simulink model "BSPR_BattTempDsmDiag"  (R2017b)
settings: Solver=FixedStepDiscrete  StartTime=0.0  StopTime=10.0  FixedStep=1  RelTol=1e-3  EnableMultiTasking=on
libraries: simulink x112

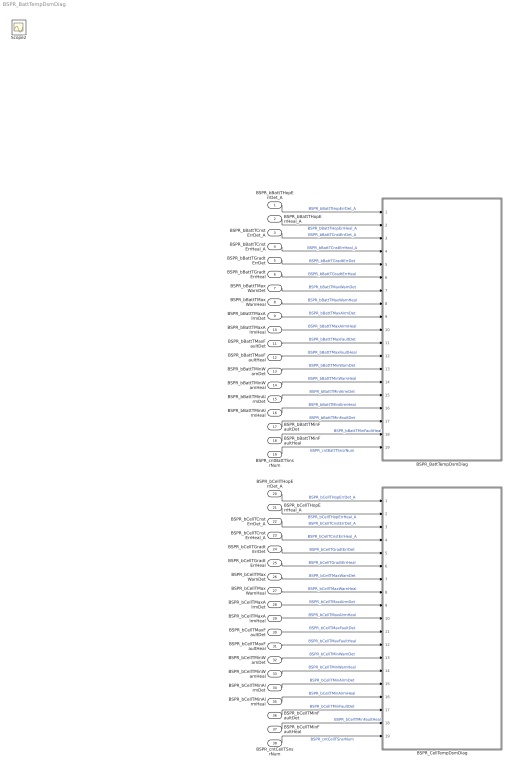
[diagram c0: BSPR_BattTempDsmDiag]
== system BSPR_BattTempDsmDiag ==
  BSPR_bBattTHopErrDet_A : Inport
  BSPR_bBattTHopErrHeal_A : Inport  Port=2
  BSPR_bBattTCnstErrDet_A : Inport  Port=3
  BSPR_bBattTCnstErrHeal_A : Inport  Port=4
  BSPR_bBattTGradtErrDet : Inport  Port=5  OutDataTypeStr=boolean
  BSPR_bBattTGradtErrHeal : Inport  Port=6  OutDataTypeStr=boolean
  BSPR_bBattTMaxWarnDet : Inport  Port=7
  BSPR_bBattTMaxWarnHeal : Inport  Port=8
  BSPR_bBattTMaxAlrmDet : Inport  Port=9
  BSPR_bBattTMaxAlrmHeal : Inport  Port=10
  BSPR_bBattTMaxFaultDet : Inport  Port=11
  BSPR_bBattTMaxFaultHeal : Inport  Port=12
  BSPR_bBattTMinWarnDet : Inport  Port=13
  BSPR_bBattTMinWarnHeal : Inport  Port=14
  BSPR_bBattTMinAlrmDet : Inport  Port=15
  BSPR_bBattTMinAlrmHeal : Inport  Port=16
  BSPR_bBattTMinFaultDet : Inport  Port=17
  BSPR_bBattTMinFaultHeal : Inport  Port=18
  BSPR_cntBattTSnsrNum : Inport  Port=19
  BSPR_bCellTHopErrDet_A : Inport  Port=20
  BSPR_bCellTHopErrHeal_A : Inport  Port=21
  BSPR_bCellTCnstErrDet_A : Inport  Port=22
  BSPR_bCellTCnstErrHeal_A : Inport  Port=23
  BSPR_bCellTGradtErrDet : Inport  Port=24  OutDataTypeStr=boolean
  BSPR_bCellTGradtErrHeal : Inport  Port=25  OutDataTypeStr=boolean
  BSPR_bCellTMaxWarnDet : Inport  Port=26
  BSPR_bCellTMaxWarnHeal : Inport  Port=27
  BSPR_bCellTMaxAlrmDet : Inport  Port=28
  BSPR_bCellTMaxAlrmHeal : Inport  Port=29
  BSPR_bCellTMaxFaultDet : Inport  Port=30
  BSPR_bCellTMaxFaultHeal : Inport  Port=31
  BSPR_bCellTMinWarnDet : Inport  Port=32
  BSPR_bCellTMinWarnHeal : Inport  Port=33
  BSPR_bCellTMinAlrmDet : Inport  Port=34
  BSPR_bCellTMinAlrmHeal : Inport  Port=35
  BSPR_bCellTMinFaultDet : Inport  Port=36
  BSPR_bCellTMinFaultHeal : Inport  Port=37
  BSPR_cntCellTSnsrNum : Inport  Port=38
  BSPR_BattTempDsmDiag : Subsystem
  BSPR_CellTempDsmDiag : Subsystem
  Scope2 : Scope
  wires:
  BSPR_bBattTMaxWarnDet/1 -> BSPR_BattTempDsmDiag/7(BSPR_bBattTMaxWarnDet)  "BSPR_bBattTMaxWarnDet"
  BSPR_bBattTMaxWarnHeal/1 -> BSPR_BattTempDsmDiag/8(BSPR_bBattTMaxWarnHeal)  "BSPR_bBattTMaxWarnHeal"
  BSPR_bBattTMaxAlrmDet/1 -> BSPR_BattTempDsmDiag/9(BSPR_bBattTMaxAlrmDet)  "BSPR_bBattTMaxAlrmDet"
  BSPR_bBattTMaxAlrmHeal/1 -> BSPR_BattTempDsmDiag/10(BSPR_bBattTMaxAlrmHeal)  "BSPR_bBattTMaxAlrmHeal"
  BSPR_bBattTMaxFaultDet/1 -> BSPR_BattTempDsmDiag/11(BSPR_bBattTMaxFaultDet)  "BSPR_bBattTMaxFaultDet"
  BSPR_bBattTMaxFaultHeal/1 -> BSPR_BattTempDsmDiag/12(BSPR_bBattTMaxFaultHeal)  "BSPR_bBattTMaxFaultHeal"
  BSPR_bBattTMinWarnDet/1 -> BSPR_BattTempDsmDiag/13(BSPR_bBattTMinWarnDet)  "BSPR_bBattTMinWarnDet"
  BSPR_bBattTMinWarnHeal/1 -> BSPR_BattTempDsmDiag/14(BSPR_bBattTMinWarnHeal)  "BSPR_bBattTMinWarnHeal"
  BSPR_bBattTMinAlrmDet/1 -> BSPR_BattTempDsmDiag/15(BSPR_bBattTMinAlrmDet)  "BSPR_bBattTMinAlrmDet"
  BSPR_bBattTMinAlrmHeal/1 -> BSPR_BattTempDsmDiag/16(BSPR_bBattTMinAlrmHeal)  "BSPR_bBattTMinAlrmHeal"
  BSPR_bBattTMinFaultDet/1 -> BSPR_BattTempDsmDiag/17(BSPR_bBattTMinFaultDet)  "BSPR_bBattTMinFaultDet"
  BSPR_bBattTMinFaultHeal/1 -> BSPR_BattTempDsmDiag/18(BSPR_bBattTMinFaultHeal)  "BSPR_bBattTMinFaultHeal"
  BSPR_bBattTCnstErrHeal_A/1 -> BSPR_BattTempDsmDiag/4(BSPR_bBattTCnstErrHeal_A)  "BSPR_bBattTCnstErrHeal_A"
  BSPR_bBattTCnstErrDet_A/1 -> BSPR_BattTempDsmDiag/3(BSPR_bBattTCnstErrDet_A)  "BSPR_bBattTCnstErrDet_A"
  BSPR_bBattTHopErrHeal_A/1 -> BSPR_BattTempDsmDiag/2(BSPR_bBattTHopErrHeal_A)  "BSPR_bBattTHopErrHeal_A"
  BSPR_bBattTHopErrDet_A/1 -> BSPR_BattTempDsmDiag/1(BSPR_bBattTHopErrDet_A)  "BSPR_bBattTHopErrDet_A"
  BSPR_bBattTGradtErrDet/1 -> BSPR_BattTempDsmDiag/5(BSPR_bBattTGradtErrDet)  "BSPR_bBattTGradtErrDet"
  BSPR_bBattTGradtErrHeal/1 -> BSPR_BattTempDsmDiag/6(BSPR_bBattTGradtErrHeal)  "BSPR_bBattTGradtErrHeal"
  BSPR_cntBattTSnsrNum/1 -> BSPR_BattTempDsmDiag/19(BSPR_cntBattTSnsrNum)  "BSPR_cntBattTSnsrNum"
  BSPR_cntCellTSnsrNum/1 -> BSPR_CellTempDsmDiag/19(BSPR_cntCellTSnsrNum)  "BSPR_cntCellTSnsrNum"
  BSPR_bCellTGradtErrHeal/1 -> BSPR_CellTempDsmDiag/6(BSPR_bCellTGradtErrHeal)  "BSPR_bCellTGradtErrHeal"
  BSPR_bCellTGradtErrDet/1 -> BSPR_CellTempDsmDiag/5(BSPR_bCellTGradtErrDet)  "BSPR_bCellTGradtErrDet"
  BSPR_bCellTHopErrDet_A/1 -> BSPR_CellTempDsmDiag/1(BSPR_bCellTHopErrDet_A)  "BSPR_bCellTHopErrDet_A"
  BSPR_bCellTHopErrHeal_A/1 -> BSPR_CellTempDsmDiag/2(BSPR_bCellTHopErrHeal_A)  "BSPR_bCellTHopErrHeal_A"
  BSPR_bCellTCnstErrDet_A/1 -> BSPR_CellTempDsmDiag/3(BSPR_bCellTCnstErrDet_A)  "BSPR_bCellTCnstErrDet_A"
  BSPR_bCellTCnstErrHeal_A/1 -> BSPR_CellTempDsmDiag/4(BSPR_bCellTCnstErrHeal_A)  "BSPR_bCellTCnstErrHeal_A"
  BSPR_bCellTMinFaultHeal/1 -> BSPR_CellTempDsmDiag/18(BSPR_bCellTMinFaultHeal)  "BSPR_bCellTMinFaultHeal"
  BSPR_bCellTMinFaultDet/1 -> BSPR_CellTempDsmDiag/17(BSPR_bCellTMinFaultDet)  "BSPR_bCellTMinFaultDet"
  BSPR_bCellTMinAlrmHeal/1 -> BSPR_CellTempDsmDiag/16(BSPR_bCellTMinAlrmHeal)  "BSPR_bCellTMinAlrmHeal"
  BSPR_bCellTMinAlrmDet/1 -> BSPR_CellTempDsmDiag/15(BSPR_bCellTMinAlrmDet)  "BSPR_bCellTMinAlrmDet"
  BSPR_bCellTMinWarnHeal/1 -> BSPR_CellTempDsmDiag/14(BSPR_bCellTMinWarnHeal)  "BSPR_bCellTMinWarnHeal"
  BSPR_bCellTMinWarnDet/1 -> BSPR_CellTempDsmDiag/13(BSPR_bCellTMinWarnDet)  "BSPR_bCellTMinWarnDet"
  BSPR_bCellTMaxFaultHeal/1 -> BSPR_CellTempDsmDiag/12(BSPR_bCellTMaxFaultHeal)  "BSPR_bCellTMaxFaultHeal"
  BSPR_bCellTMaxFaultDet/1 -> BSPR_CellTempDsmDiag/11(BSPR_bCellTMaxFaultDet)  "BSPR_bCellTMaxFaultDet"
  BSPR_bCellTMaxAlrmHeal/1 -> BSPR_CellTempDsmDiag/10(BSPR_bCellTMaxAlrmHeal)  "BSPR_bCellTMaxAlrmHeal"
  BSPR_bCellTMaxAlrmDet/1 -> BSPR_CellTempDsmDiag/9(BSPR_bCellTMaxAlrmDet)  "BSPR_bCellTMaxAlrmDet"
  BSPR_bCellTMaxWarnHeal/1 -> BSPR_CellTempDsmDiag/8(BSPR_bCellTMaxWarnHeal)  "BSPR_bCellTMaxWarnHeal"
  BSPR_bCellTMaxWarnDet/1 -> BSPR_CellTempDsmDiag/7(BSPR_bCellTMaxWarnDet)  "BSPR_bCellTMaxWarnDet"

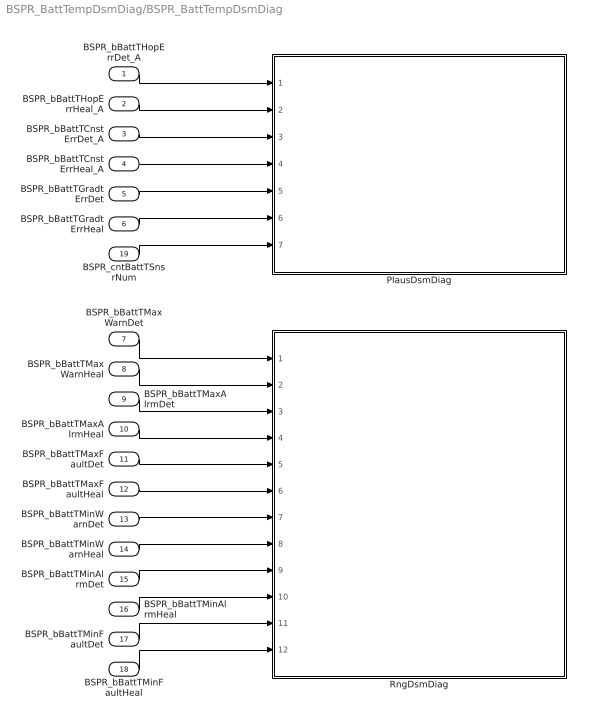
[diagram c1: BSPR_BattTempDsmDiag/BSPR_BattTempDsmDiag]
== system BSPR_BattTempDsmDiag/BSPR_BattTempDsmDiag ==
  BSPR_bBattTHopErrDet_A : Inport
  BSPR_bBattTHopErrHeal_A : Inport  Port=2
  BSPR_bBattTCnstErrDet_A : Inport  Port=3
  BSPR_bBattTCnstErrHeal_A : Inport  Port=4
  BSPR_bBattTGradtErrDet : Inport  Port=5  OutDataTypeStr=boolean
  BSPR_bBattTGradtErrHeal : Inport  Port=6  OutDataTypeStr=boolean
  BSPR_bBattTMaxWarnDet : Inport  Port=7
  BSPR_bBattTMaxWarnHeal : Inport  Port=8
  BSPR_bBattTMaxAlrmDet : Inport  Port=9
  BSPR_bBattTMaxAlrmHeal : Inport  Port=10
  BSPR_bBattTMaxFaultDet : Inport  Port=11
  BSPR_bBattTMaxFaultHeal : Inport  Port=12
  BSPR_bBattTMinWarnDet : Inport  Port=13
  BSPR_bBattTMinWarnHeal : Inport  Port=14
  BSPR_bBattTMinAlrmDet : Inport  Port=15
  BSPR_bBattTMinAlrmHeal : Inport  Port=16
  BSPR_bBattTMinFaultDet : Inport  Port=17
  BSPR_bBattTMinFaultHeal : Inport  Port=18
  BSPR_cntBattTSnsrNum : Inport  Port=19
  PlausDsmDiag : Subsystem
  RngDsmDiag : Subsystem
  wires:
  BSPR_bBattTMaxWarnDet/1 -> RngDsmDiag/1(BSPR_bBattTMaxWarnDet)
  BSPR_bBattTMaxWarnHeal/1 -> RngDsmDiag/2(BSPR_bBattTMaxWarnHeal)
  BSPR_bBattTMaxAlrmDet/1 -> RngDsmDiag/3(BSPR_bBattTMaxAlrmDet)
  BSPR_bBattTMaxAlrmHeal/1 -> RngDsmDiag/4(BSPR_bBattTMaxAlrmHeal)
  BSPR_bBattTMaxFaultDet/1 -> RngDsmDiag/5(BSPR_bBattTMaxFaultDet)
  BSPR_bBattTMaxFaultHeal/1 -> RngDsmDiag/6(BSPR_bBattTMaxFaultHeal)
  BSPR_bBattTMinWarnDet/1 -> RngDsmDiag/7(BSPR_bBattTMinWarnDet)
  BSPR_bBattTMinWarnHeal/1 -> RngDsmDiag/8(BSPR_bBattTMinWarnHeal)
  BSPR_bBattTMinAlrmDet/1 -> RngDsmDiag/9(BSPR_bBattTMinAlrmDet)
  BSPR_bBattTMinAlrmHeal/1 -> RngDsmDiag/10(BSPR_bBattTMinAlrmHeal)
  BSPR_bBattTMinFaultDet/1 -> RngDsmDiag/11(BSPR_bBattTMinFaultDet)
  BSPR_bBattTMinFaultHeal/1 -> RngDsmDiag/12(BSPR_bBattTMinFaultHeal)
  BSPR_bBattTCnstErrHeal_A/1 -> PlausDsmDiag/4(BSPR_bBattTCnstErrHeal_A)
  BSPR_bBattTCnstErrDet_A/1 -> PlausDsmDiag/3(BSPR_bBattTCnstErrDet_A)
  BSPR_bBattTHopErrHeal_A/1 -> PlausDsmDiag/2(BSPR_bBattTHopErrHeal_A)
  BSPR_bBattTHopErrDet_A/1 -> PlausDsmDiag/1(BSPR_bBattTHopErrDet_A)
  BSPR_bBattTGradtErrHeal/1 -> PlausDsmDiag/6(BSPR_bBattTGradtErrHeal)
  BSPR_bBattTGradtErrDet/1 -> PlausDsmDiag/5(BSPR_bBattTGradtErrDet)
  BSPR_cntBattTSnsrNum/1 -> PlausDsmDiag/7(BSPR_cntBattTSnsrNum)

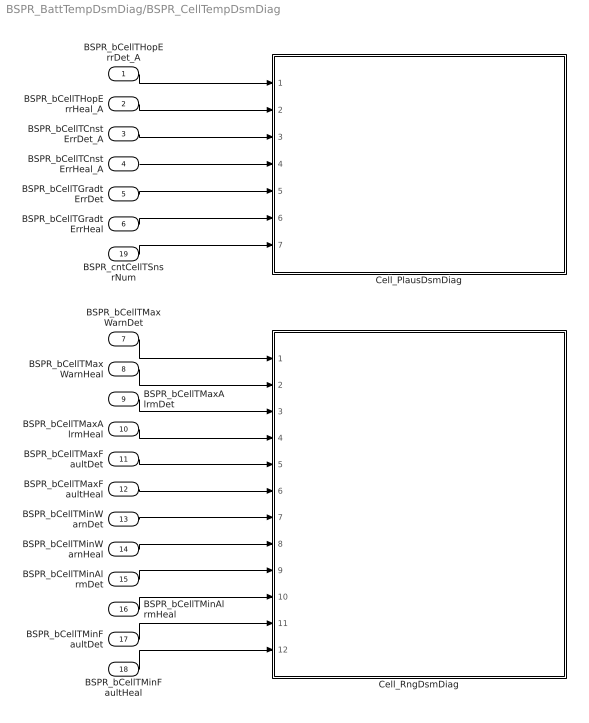
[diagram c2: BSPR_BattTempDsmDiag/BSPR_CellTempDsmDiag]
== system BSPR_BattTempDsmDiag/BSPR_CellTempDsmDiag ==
  BSPR_bCellTHopErrDet_A : Inport
  BSPR_bCellTHopErrHeal_A : Inport  Port=2
  BSPR_bCellTCnstErrDet_A : Inport  Port=3
  BSPR_bCellTCnstErrHeal_A : Inport  Port=4
  BSPR_bCellTGradtErrDet : Inport  Port=5  OutDataTypeStr=boolean
  BSPR_bCellTGradtErrHeal : Inport  Port=6  OutDataTypeStr=boolean
  BSPR_bCellTMaxWarnDet : Inport  Port=7
  BSPR_bCellTMaxWarnHeal : Inport  Port=8
  BSPR_bCellTMaxAlrmDet : Inport  Port=9
  BSPR_bCellTMaxAlrmHeal : Inport  Port=10
  BSPR_bCellTMaxFaultDet : Inport  Port=11
  BSPR_bCellTMaxFaultHeal : Inport  Port=12
  BSPR_bCellTMinWarnDet : Inport  Port=13
  BSPR_bCellTMinWarnHeal : Inport  Port=14
  BSPR_bCellTMinAlrmDet : Inport  Port=15
  BSPR_bCellTMinAlrmHeal : Inport  Port=16
  BSPR_bCellTMinFaultDet : Inport  Port=17
  BSPR_bCellTMinFaultHeal : Inport  Port=18
  BSPR_cntCellTSnsrNum : Inport  Port=19
  Cell_PlausDsmDiag : Subsystem
  Cell_RngDsmDiag : Subsystem
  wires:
  BSPR_cntCellTSnsrNum/1 -> Cell_PlausDsmDiag/7(BSPR_cntCellTSnsrNum)
  BSPR_bCellTGradtErrDet/1 -> Cell_PlausDsmDiag/5(BSPR_bCellTGradtErrDet)
  BSPR_bCellTGradtErrHeal/1 -> Cell_PlausDsmDiag/6(BSPR_bCellTGradtErrHeal)
  BSPR_bCellTHopErrDet_A/1 -> Cell_PlausDsmDiag/1(BSPR_bCellTHopErrDet_A)
  BSPR_bCellTHopErrHeal_A/1 -> Cell_PlausDsmDiag/2(BSPR_bCellTHopErrHeal_A)
  BSPR_bCellTCnstErrDet_A/1 -> Cell_PlausDsmDiag/3(BSPR_bCellTCnstErrDet_A)
  BSPR_bCellTCnstErrHeal_A/1 -> Cell_PlausDsmDiag/4(BSPR_bCellTCnstErrHeal_A)
  BSPR_bCellTMinFaultHeal/1 -> Cell_RngDsmDiag/12(BSPR_bCellTMinFaultHeal)
  BSPR_bCellTMinFaultDet/1 -> Cell_RngDsmDiag/11(BSPR_bCellTMinFaultDet)
  BSPR_bCellTMinAlrmHeal/1 -> Cell_RngDsmDiag/10(BSPR_bCellTMinAlrmHeal)
  BSPR_bCellTMinAlrmDet/1 -> Cell_RngDsmDiag/9(BSPR_bCellTMinAlrmDet)
  BSPR_bCellTMinWarnHeal/1 -> Cell_RngDsmDiag/8(BSPR_bCellTMinWarnHeal)
  BSPR_bCellTMinWarnDet/1 -> Cell_RngDsmDiag/7(BSPR_bCellTMinWarnDet)
  BSPR_bCellTMaxFaultHeal/1 -> Cell_RngDsmDiag/6(BSPR_bCellTMaxFaultHeal)
  BSPR_bCellTMaxFaultDet/1 -> Cell_RngDsmDiag/5(BSPR_bCellTMaxFaultDet)
  BSPR_bCellTMaxAlrmHeal/1 -> Cell_RngDsmDiag/4(BSPR_bCellTMaxAlrmHeal)
  BSPR_bCellTMaxAlrmDet/1 -> Cell_RngDsmDiag/3(BSPR_bCellTMaxAlrmDet)
  BSPR_bCellTMaxWarnHeal/1 -> Cell_RngDsmDiag/2(BSPR_bCellTMaxWarnHeal)
  BSPR_bCellTMaxWarnDet/1 -> Cell_RngDsmDiag/1(BSPR_bCellTMaxWarnDet)

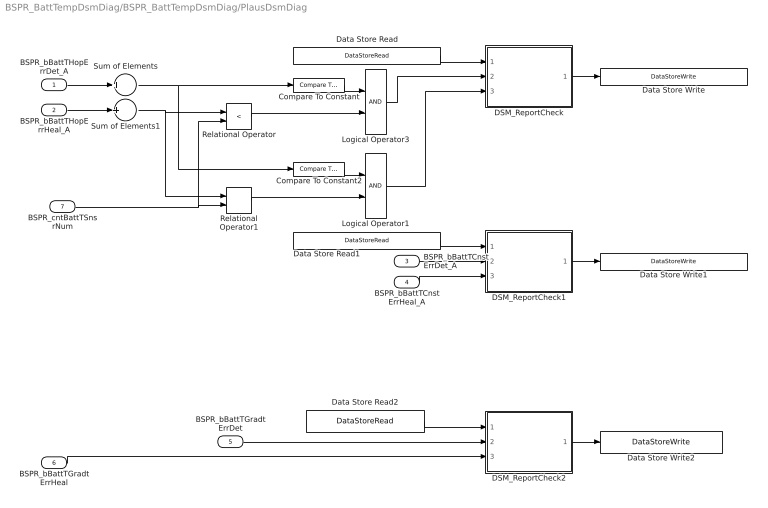
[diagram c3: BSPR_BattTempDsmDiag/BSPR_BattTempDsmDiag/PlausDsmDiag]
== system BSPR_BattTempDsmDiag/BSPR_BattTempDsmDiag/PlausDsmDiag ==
  BSPR_bBattTHopErrDet_A : Inport
  BSPR_bBattTHopErrHeal_A : Inport  Port=2
  BSPR_bBattTCnstErrDet_A : Inport  Port=3
  BSPR_bBattTCnstErrHeal_A : Inport  Port=4
  BSPR_bBattTGradtErrDet : Inport  Port=5
  BSPR_bBattTGradtErrHeal : Inport  Port=6
  BSPR_cntBattTSnsrNum : Inport  Port=7
  Compare To Constant : simulink/Logic and Bit Operations/Compare To Constant  relop=>  const=0  OutDataTypeStr=boolean
  Compare To Constant2 : simulink/Logic and Bit Operations/Compare To Constant  relop===  const=0  OutDataTypeStr=boolean
  DSM_ReportCheck : Subsystem  TreatAsAtomicUnit=on  RTWFcnName=DSM_ReportCheck  RTWFileName=SrvLib
  DSM_ReportCheck1 : Subsystem  TreatAsAtomicUnit=on  RTWFcnName=DSM_ReportCheck  RTWFileName=SrvLib
  DSM_ReportCheck2 : Subsystem  TreatAsAtomicUnit=on  RTWFcnName=DSM_ReportCheck  RTWFileName=SrvLib
  Data Store Read : DataStoreRead  DataStoreName=DFC_BattTHopMax
  Data Store Read1 : DataStoreRead  DataStoreName=DFC_BattTCnstMax
  Data Store Read2 : DataStoreRead  DataStoreName=DFC_BattTGradtMax
  Data Store Write : DataStoreWrite  DataStoreName=DFC_BattTHopMax
  Data Store Write1 : DataStoreWrite  DataStoreName=DFC_BattTCnstMax
  Data Store Write2 : DataStoreWrite  DataStoreName=DFC_BattTGradtMax
  Logical Operator1 : Logic  AllPortsSameDT=off  OutDataTypeStr=boolean
  Logical Operator3 : Logic  AllPortsSameDT=off  OutDataTypeStr=boolean
  Relational Operator : RelationalOperator  Operator=<  OutDataTypeStr=boolean  RndMeth=Simplest
  Relational Operator1 : RelationalOperator  Operator===  OutDataTypeStr=boolean  RndMeth=Simplest
  Sum of Elements : Sum  Inputs=+
  Sum of Elements1 : Sum  Inputs=+
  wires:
  Data Store Read/1 -> DSM_ReportCheck/1(Dfc_id_nv)
  DSM_ReportCheck/1(Dfc_id) -> Data Store Write/1
  DSM_ReportCheck1/1(Dfc_id) -> Data Store Write1/1
  Compare To Constant/1 -> Logical Operator3/1
  Sum of Elements/1 -> Compare To Constant/1, Compare To Constant2/1
  Sum of Elements1/1 -> Relational Operator1/1, Relational Operator/1
  Relational Operator/1 -> Logical Operator3/2
  Logical Operator3/1 -> DSM_ReportCheck/2(Err)
  Compare To Constant2/1 -> Logical Operator1/1
  Relational Operator1/1 -> Logical Operator1/2
  Logical Operator1/1 -> DSM_ReportCheck/3(Heal)
  BSPR_bBattTHopErrDet_A/1 -> Sum of Elements/1
  BSPR_bBattTHopErrHeal_A/1 -> Sum of Elements1/1
  BSPR_bBattTCnstErrDet_A/1 -> DSM_ReportCheck1/2(Err)
  BSPR_bBattTCnstErrHeal_A/1 -> DSM_ReportCheck1/3(Heal)
  Data Store Read1/1 -> DSM_ReportCheck1/1(Dfc_id_nv)
  BSPR_bBattTGradtErrHeal/1 -> DSM_ReportCheck2/3(Heal)
  BSPR_bBattTGradtErrDet/1 -> DSM_ReportCheck2/2(Err)
  Data Store Read2/1 -> DSM_ReportCheck2/1(Dfc_id_nv)
  DSM_ReportCheck2/1(Dfc_id) -> Data Store Write2/1
  BSPR_cntBattTSnsrNum/1 -> Relational Operator/2, Relational Operator1/2

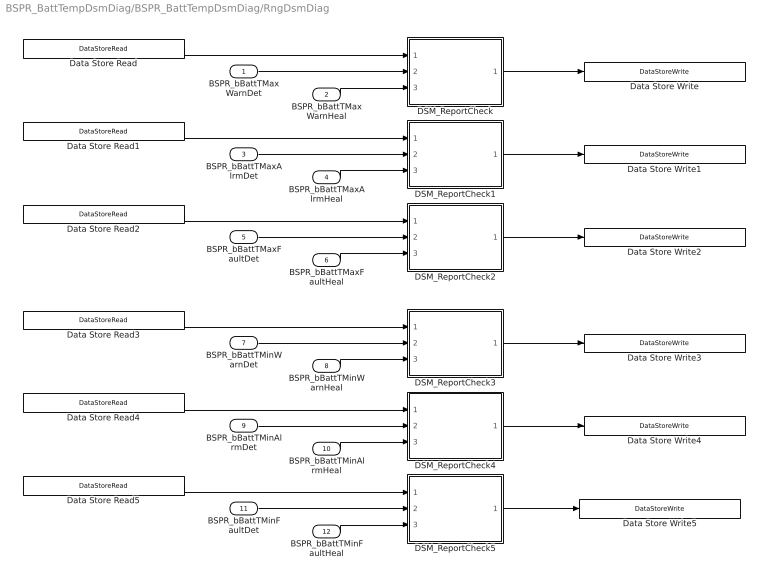
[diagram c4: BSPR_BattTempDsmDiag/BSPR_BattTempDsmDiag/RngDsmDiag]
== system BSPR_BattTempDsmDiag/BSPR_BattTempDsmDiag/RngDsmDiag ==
  BSPR_bBattTMaxWarnDet : Inport
  BSPR_bBattTMaxWarnHeal : Inport  Port=2
  BSPR_bBattTMaxAlrmDet : Inport  Port=3
  BSPR_bBattTMaxAlrmHeal : Inport  Port=4
  BSPR_bBattTMaxFaultDet : Inport  Port=5
  BSPR_bBattTMaxFaultHeal : Inport  Port=6
  BSPR_bBattTMinWarnDet : Inport  Port=7
  BSPR_bBattTMinWarnHeal : Inport  Port=8
  BSPR_bBattTMinAlrmDet : Inport  Port=9
  BSPR_bBattTMinAlrmHeal : Inport  Port=10
  BSPR_bBattTMinFaultDet : Inport  Port=11
  BSPR_bBattTMinFaultHeal : Inport  Port=12
  DSM_ReportCheck : Subsystem  TreatAsAtomicUnit=on  RTWFcnName=DSM_ReportCheck  RTWFileName=SrvLib
  DSM_ReportCheck1 : Subsystem  TreatAsAtomicUnit=on  RTWFcnName=DSM_ReportCheck  RTWFileName=SrvLib
  DSM_ReportCheck2 : Subsystem  TreatAsAtomicUnit=on  RTWFcnName=DSM_ReportCheck  RTWFileName=SrvLib
  DSM_ReportCheck3 : Subsystem  TreatAsAtomicUnit=on  RTWFcnName=DSM_ReportCheck  RTWFileName=SrvLib
  DSM_ReportCheck4 : Subsystem  TreatAsAtomicUnit=on  RTWFcnName=DSM_ReportCheck  RTWFileName=SrvLib
  DSM_ReportCheck5 : Subsystem  TreatAsAtomicUnit=on  RTWFcnName=DSM_ReportCheck  RTWFileName=SrvLib
  Data Store Read : DataStoreRead  DataStoreName=DFC_BattTWarnMax
  Data Store Read1 : DataStoreRead  DataStoreName=DFC_BattTAlrmMax
  Data Store Read2 : DataStoreRead  DataStoreName=DFC_BattTFaultMax
  Data Store Read3 : DataStoreRead  DataStoreName=DFC_BattTWarnMin
  Data Store Read4 : DataStoreRead  DataStoreName=DFC_BattTAlrmMin
  Data Store Read5 : DataStoreRead  DataStoreName=DFC_BattTFaultMin
  Data Store Write : DataStoreWrite  DataStoreName=DFC_BattTWarnMax
  Data Store Write1 : DataStoreWrite  DataStoreName=DFC_BattTAlrmMax
  Data Store Write2 : DataStoreWrite  DataStoreName=DFC_BattTFaultMax
  Data Store Write3 : DataStoreWrite  DataStoreName=DFC_BattTWarnMin
  Data Store Write4 : DataStoreWrite  DataStoreName=DFC_BattTAlrmMin
  Data Store Write5 : DataStoreWrite  DataStoreName=DFC_BattTFaultMin
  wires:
  Data Store Read/1 -> DSM_ReportCheck/1(Dfc_id_nv)
  BSPR_bBattTMaxWarnDet/1 -> DSM_ReportCheck/2(Err)
  BSPR_bBattTMaxWarnHeal/1 -> DSM_ReportCheck/3(Heal)
  Data Store Read1/1 -> DSM_ReportCheck1/1(Dfc_id_nv)
  BSPR_bBattTMaxAlrmDet/1 -> DSM_ReportCheck1/2(Err)
  BSPR_bBattTMaxAlrmHeal/1 -> DSM_ReportCheck1/3(Heal)
  Data Store Read2/1 -> DSM_ReportCheck2/1(Dfc_id_nv)
  BSPR_bBattTMaxFaultDet/1 -> DSM_ReportCheck2/2(Err)
  BSPR_bBattTMaxFaultHeal/1 -> DSM_ReportCheck2/3(Heal)
  Data Store Read3/1 -> DSM_ReportCheck3/1(Dfc_id_nv)
  BSPR_bBattTMinWarnDet/1 -> DSM_ReportCheck3/2(Err)
  BSPR_bBattTMinWarnHeal/1 -> DSM_ReportCheck3/3(Heal)
  Data Store Read5/1 -> DSM_ReportCheck5/1(Dfc_id_nv)
  Data Store Read4/1 -> DSM_ReportCheck4/1(Dfc_id_nv)
  BSPR_bBattTMinAlrmDet/1 -> DSM_ReportCheck4/2(Err)
  BSPR_bBattTMinAlrmHeal/1 -> DSM_ReportCheck4/3(Heal)
  BSPR_bBattTMinFaultDet/1 -> DSM_ReportCheck5/2(Err)
  BSPR_bBattTMinFaultHeal/1 -> DSM_ReportCheck5/3(Heal)
  DSM_ReportCheck/1(Dfc_id) -> Data Store Write/1
  DSM_ReportCheck1/1(Dfc_id) -> Data Store Write1/1
  DSM_ReportCheck2/1(Dfc_id) -> Data Store Write2/1
  DSM_ReportCheck3/1(Dfc_id) -> Data Store Write3/1
  DSM_ReportCheck4/1(Dfc_id) -> Data Store Write4/1
  DSM_ReportCheck5/1(Dfc_id) -> Data Store Write5/1

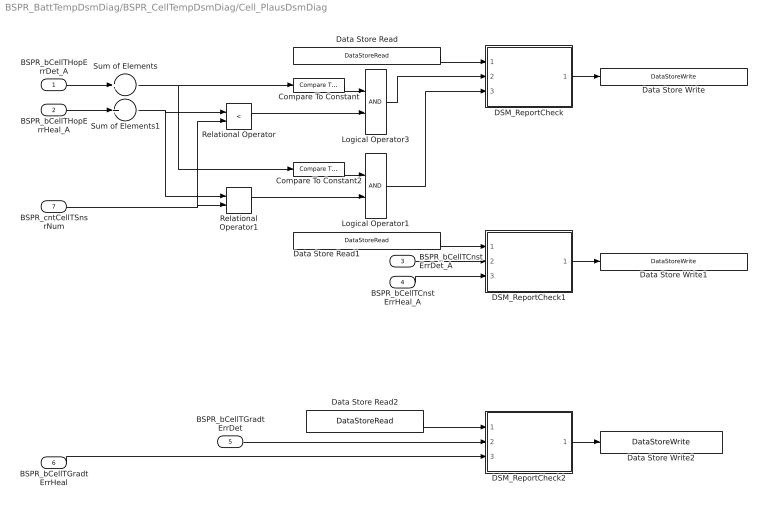
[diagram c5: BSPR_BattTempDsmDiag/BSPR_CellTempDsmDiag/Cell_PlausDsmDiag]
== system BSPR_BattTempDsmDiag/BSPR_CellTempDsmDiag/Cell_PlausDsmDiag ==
  BSPR_bCellTHopErrDet_A : Inport
  BSPR_bCellTHopErrHeal_A : Inport  Port=2
  BSPR_bCellTCnstErrDet_A : Inport  Port=3
  BSPR_bCellTCnstErrHeal_A : Inport  Port=4
  BSPR_bCellTGradtErrDet : Inport  Port=5
  BSPR_bCellTGradtErrHeal : Inport  Port=6
  BSPR_cntCellTSnsrNum : Inport  Port=7
  Compare To Constant : simulink/Logic and Bit Operations/Compare To Constant  relop=>  const=0  OutDataTypeStr=boolean
  Compare To Constant2 : simulink/Logic and Bit Operations/Compare To Constant  relop===  const=0  OutDataTypeStr=boolean
  DSM_ReportCheck : Subsystem  TreatAsAtomicUnit=on  RTWFcnName=DSM_ReportCheck  RTWFileName=SrvLib
  DSM_ReportCheck1 : Subsystem  TreatAsAtomicUnit=on  RTWFcnName=DSM_ReportCheck  RTWFileName=SrvLib
  DSM_ReportCheck2 : Subsystem  TreatAsAtomicUnit=on  RTWFcnName=DSM_ReportCheck  RTWFileName=SrvLib
  Data Store Read : DataStoreRead  DataStoreName=DFC_CellTHopMax
  Data Store Read1 : DataStoreRead  DataStoreName=DFC_CellTCnstMax
  Data Store Read2 : DataStoreRead  DataStoreName=DFC_CellTGradtMax
  Data Store Write : DataStoreWrite  DataStoreName=DFC_CellTHopMax
  Data Store Write1 : DataStoreWrite  DataStoreName=DFC_CellTCnstMax
  Data Store Write2 : DataStoreWrite  DataStoreName=DFC_CellTGradtMax
  Logical Operator1 : Logic  AllPortsSameDT=off  OutDataTypeStr=boolean
  Logical Operator3 : Logic  AllPortsSameDT=off  OutDataTypeStr=boolean
  Relational Operator : RelationalOperator  Operator=<  OutDataTypeStr=boolean  RndMeth=Simplest
  Relational Operator1 : RelationalOperator  Operator===  OutDataTypeStr=boolean  RndMeth=Simplest
  Sum of Elements : Sum  Inputs=+
  Sum of Elements1 : Sum  Inputs=+
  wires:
  BSPR_cntCellTSnsrNum/1 -> Relational Operator1/2, Relational Operator/2
  DSM_ReportCheck2/1(Dfc_id) -> Data Store Write2/1
  Data Store Read2/1 -> DSM_ReportCheck2/1(Dfc_id_nv)
  BSPR_bCellTGradtErrDet/1 -> DSM_ReportCheck2/2(Err)
  BSPR_bCellTGradtErrHeal/1 -> DSM_ReportCheck2/3(Heal)
  Data Store Read1/1 -> DSM_ReportCheck1/1(Dfc_id_nv)
  BSPR_bCellTCnstErrHeal_A/1 -> DSM_ReportCheck1/3(Heal)
  BSPR_bCellTCnstErrDet_A/1 -> DSM_ReportCheck1/2(Err)
  BSPR_bCellTHopErrHeal_A/1 -> Sum of Elements1/1
  BSPR_bCellTHopErrDet_A/1 -> Sum of Elements/1
  Logical Operator1/1 -> DSM_ReportCheck/3(Heal)
  Relational Operator1/1 -> Logical Operator1/2
  Compare To Constant2/1 -> Logical Operator1/1
  Logical Operator3/1 -> DSM_ReportCheck/2(Err)
  Relational Operator/1 -> Logical Operator3/2
  Sum of Elements1/1 -> Relational Operator/1, Relational Operator1/1
  Sum of Elements/1 -> Compare To Constant2/1, Compare To Constant/1
  Compare To Constant/1 -> Logical Operator3/1
  DSM_ReportCheck1/1(Dfc_id) -> Data Store Write1/1
  DSM_ReportCheck/1(Dfc_id) -> Data Store Write/1
  Data Store Read/1 -> DSM_ReportCheck/1(Dfc_id_nv)

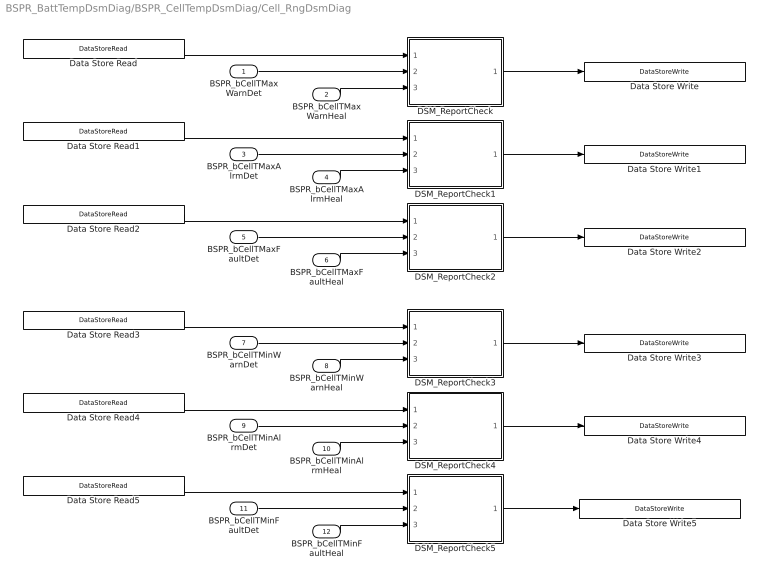
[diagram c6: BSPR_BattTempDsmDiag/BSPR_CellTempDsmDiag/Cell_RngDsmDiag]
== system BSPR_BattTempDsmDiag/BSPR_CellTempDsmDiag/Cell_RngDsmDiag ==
  BSPR_bCellTMaxWarnDet : Inport
  BSPR_bCellTMaxWarnHeal : Inport  Port=2
  BSPR_bCellTMaxAlrmDet : Inport  Port=3
  BSPR_bCellTMaxAlrmHeal : Inport  Port=4
  BSPR_bCellTMaxFaultDet : Inport  Port=5
  BSPR_bCellTMaxFaultHeal : Inport  Port=6
  BSPR_bCellTMinWarnDet : Inport  Port=7
  BSPR_bCellTMinWarnHeal : Inport  Port=8
  BSPR_bCellTMinAlrmDet : Inport  Port=9
  BSPR_bCellTMinAlrmHeal : Inport  Port=10
  BSPR_bCellTMinFaultDet : Inport  Port=11
  BSPR_bCellTMinFaultHeal : Inport  Port=12
  DSM_ReportCheck : Subsystem  TreatAsAtomicUnit=on  RTWFcnName=DSM_ReportCheck  RTWFileName=SrvLib
  DSM_ReportCheck1 : Subsystem  TreatAsAtomicUnit=on  RTWFcnName=DSM_ReportCheck  RTWFileName=SrvLib
  DSM_ReportCheck2 : Subsystem  TreatAsAtomicUnit=on  RTWFcnName=DSM_ReportCheck  RTWFileName=SrvLib
  DSM_ReportCheck3 : Subsystem  TreatAsAtomicUnit=on  RTWFcnName=DSM_ReportCheck  RTWFileName=SrvLib
  DSM_ReportCheck4 : Subsystem  TreatAsAtomicUnit=on  RTWFcnName=DSM_ReportCheck  RTWFileName=SrvLib
  DSM_ReportCheck5 : Subsystem  TreatAsAtomicUnit=on  RTWFcnName=DSM_ReportCheck  RTWFileName=SrvLib
  Data Store Read : DataStoreRead  DataStoreName=DFC_CellTWarnMax
  Data Store Read1 : DataStoreRead  DataStoreName=DFC_CellTAlrmMax
  Data Store Read2 : DataStoreRead  DataStoreName=DFC_CellTFaultMax
  Data Store Read3 : DataStoreRead  DataStoreName=DFC_CellTWarnMin
  Data Store Read4 : DataStoreRead  DataStoreName=DFC_CellTAlrmMin
  Data Store Read5 : DataStoreRead  DataStoreName=DFC_CellTFaultMin
  Data Store Write : DataStoreWrite  DataStoreName=DFC_CellTWarnMax
  Data Store Write1 : DataStoreWrite  DataStoreName=DFC_CellTAlrmMax
  Data Store Write2 : DataStoreWrite  DataStoreName=DFC_CellTFaultMax
  Data Store Write3 : DataStoreWrite  DataStoreName=DFC_CellTWarnMin
  Data Store Write4 : DataStoreWrite  DataStoreName=DFC_CellTAlrmMin
  Data Store Write5 : DataStoreWrite  DataStoreName=DFC_CellTFaultMin
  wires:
  DSM_ReportCheck5/1(Dfc_id) -> Data Store Write5/1
  DSM_ReportCheck4/1(Dfc_id) -> Data Store Write4/1
  DSM_ReportCheck3/1(Dfc_id) -> Data Store Write3/1
  DSM_ReportCheck2/1(Dfc_id) -> Data Store Write2/1
  DSM_ReportCheck1/1(Dfc_id) -> Data Store Write1/1
  DSM_ReportCheck/1(Dfc_id) -> Data Store Write/1
  BSPR_bCellTMinFaultHeal/1 -> DSM_ReportCheck5/3(Heal)
  BSPR_bCellTMinFaultDet/1 -> DSM_ReportCheck5/2(Err)
  BSPR_bCellTMinAlrmHeal/1 -> DSM_ReportCheck4/3(Heal)
  BSPR_bCellTMinAlrmDet/1 -> DSM_ReportCheck4/2(Err)
  Data Store Read4/1 -> DSM_ReportCheck4/1(Dfc_id_nv)
  Data Store Read5/1 -> DSM_ReportCheck5/1(Dfc_id_nv)
  BSPR_bCellTMinWarnHeal/1 -> DSM_ReportCheck3/3(Heal)
  BSPR_bCellTMinWarnDet/1 -> DSM_ReportCheck3/2(Err)
  Data Store Read3/1 -> DSM_ReportCheck3/1(Dfc_id_nv)
  BSPR_bCellTMaxFaultHeal/1 -> DSM_ReportCheck2/3(Heal)
  BSPR_bCellTMaxFaultDet/1 -> DSM_ReportCheck2/2(Err)
  Data Store Read2/1 -> DSM_ReportCheck2/1(Dfc_id_nv)
  BSPR_bCellTMaxAlrmHeal/1 -> DSM_ReportCheck1/3(Heal)
  BSPR_bCellTMaxAlrmDet/1 -> DSM_ReportCheck1/2(Err)
  Data Store Read1/1 -> DSM_ReportCheck1/1(Dfc_id_nv)
  BSPR_bCellTMaxWarnHeal/1 -> DSM_ReportCheck/3(Heal)
  BSPR_bCellTMaxWarnDet/1 -> DSM_ReportCheck/2(Err)
  Data Store Read/1 -> DSM_ReportCheck/1(Dfc_id_nv)

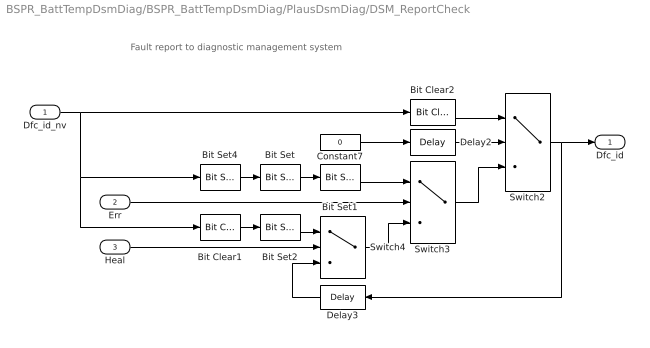
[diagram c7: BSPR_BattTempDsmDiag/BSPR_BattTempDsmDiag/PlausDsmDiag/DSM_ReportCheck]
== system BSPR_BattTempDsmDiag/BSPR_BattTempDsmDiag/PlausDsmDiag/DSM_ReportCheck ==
  note: Fault report to diagnostic management system
  Dfc_id_nv : Inport  OutDataTypeStr=uint8
  Err : Inport  Port=2
  Heal : Inport  Port=3
  Bit Clear1 : simulink/Logic and Bit Operations/Bit Clear  iBit=4
  Bit Clear2 : simulink/Logic and Bit Operations/Bit Clear  iBit=3
  Bit Set : simulink/Logic and Bit Operations/Bit Set  iBit=4
  Bit Set1 : simulink/Logic and Bit Operations/Bit Set  iBit=3
  Bit Set2 : simulink/Logic and Bit Operations/Bit Set  iBit=3
  Bit Set4 : simulink/Logic and Bit Operations/Bit Set  iBit=7
  Constant7 : Constant  Value=0  OutDataTypeStr=boolean
  Delay2 : Delay  DelayLength=1  InitialCondition=1
  Delay3 : Delay  DelayLength=1  InitialCondition=0
  Switch2 : Switch  Criteria=u2 ~= 0
  Switch3 : Switch  Criteria=u2 ~= 0
  Switch4 : Switch  Criteria=u2 ~= 0
  Dfc_id : Outport  OutDataTypeStr=uint8
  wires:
  Dfc_id_nv/1 -> Bit Clear2/1, Bit Set4/1, Bit Clear1/1
  Bit Set4/1 -> Bit Set/1
  Constant7/1 -> Delay2/1
  Delay2/1 -> Switch2/2
  Switch3/1 -> Switch2/3
  Bit Clear2/1 -> Switch2/1
  Switch2/1 -> Delay3/1, Dfc_id/1
  Bit Set1/1 -> Switch3/1
  Bit Set/1 -> Bit Set1/1
  Switch4/1 -> Switch3/3
  Err/1 -> Switch3/2
  Bit Set2/1 -> Switch4/1
  Bit Clear1/1 -> Bit Set2/1
  Delay3/1 -> Switch4/3
  Heal/1 -> Switch4/2

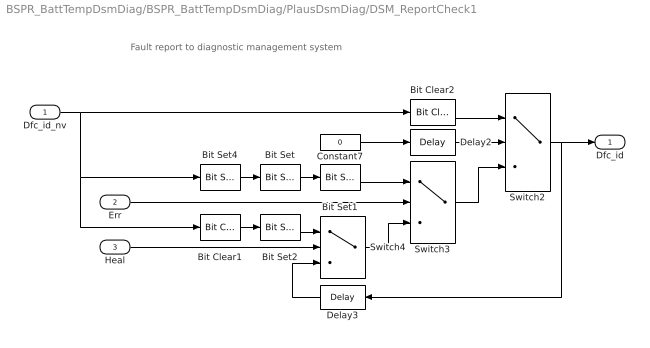
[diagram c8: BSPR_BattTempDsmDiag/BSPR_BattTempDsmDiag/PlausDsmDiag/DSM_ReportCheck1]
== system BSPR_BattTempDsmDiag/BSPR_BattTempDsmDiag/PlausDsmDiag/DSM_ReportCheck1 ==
  note: Fault report to diagnostic management system
  Dfc_id_nv : Inport  OutDataTypeStr=uint8
  Err : Inport  Port=2
  Heal : Inport  Port=3
  Bit Clear1 : simulink/Logic and Bit Operations/Bit Clear  iBit=4
  Bit Clear2 : simulink/Logic and Bit Operations/Bit Clear  iBit=3
  Bit Set : simulink/Logic and Bit Operations/Bit Set  iBit=4
  Bit Set1 : simulink/Logic and Bit Operations/Bit Set  iBit=3
  Bit Set2 : simulink/Logic and Bit Operations/Bit Set  iBit=3
  Bit Set4 : simulink/Logic and Bit Operations/Bit Set  iBit=7
  Constant7 : Constant  Value=0  OutDataTypeStr=boolean
  Delay2 : Delay  DelayLength=1  InitialCondition=1
  Delay3 : Delay  DelayLength=1  InitialCondition=0
  Switch2 : Switch  Criteria=u2 ~= 0
  Switch3 : Switch  Criteria=u2 ~= 0
  Switch4 : Switch  Criteria=u2 ~= 0
  Dfc_id : Outport  OutDataTypeStr=uint8
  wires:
  Heal/1 -> Switch4/2
  Delay3/1 -> Switch4/3
  Bit Clear1/1 -> Bit Set2/1
  Bit Set2/1 -> Switch4/1
  Err/1 -> Switch3/2
  Switch4/1 -> Switch3/3
  Bit Set/1 -> Bit Set1/1
  Bit Set1/1 -> Switch3/1
  Switch2/1 -> Dfc_id/1, Delay3/1
  Bit Clear2/1 -> Switch2/1
  Switch3/1 -> Switch2/3
  Delay2/1 -> Switch2/2
  Constant7/1 -> Delay2/1
  Bit Set4/1 -> Bit Set/1
  Dfc_id_nv/1 -> Bit Clear1/1, Bit Set4/1, Bit Clear2/1

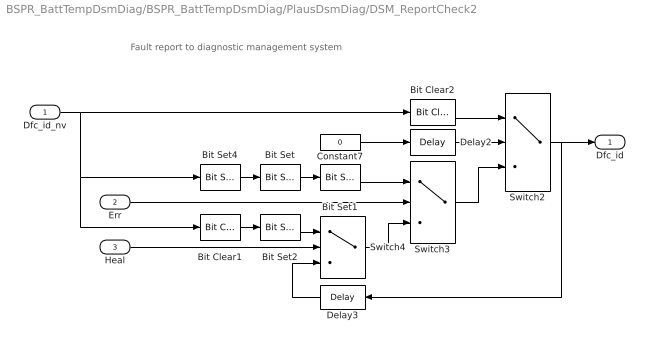
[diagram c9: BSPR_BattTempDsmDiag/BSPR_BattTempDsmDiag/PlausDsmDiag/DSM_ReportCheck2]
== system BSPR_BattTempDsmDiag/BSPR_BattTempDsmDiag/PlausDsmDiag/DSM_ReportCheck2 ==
  note: Fault report to diagnostic management system
  Dfc_id_nv : Inport  OutDataTypeStr=uint8
  Err : Inport  Port=2
  Heal : Inport  Port=3
  Bit Clear1 : simulink/Logic and Bit Operations/Bit Clear  iBit=4
  Bit Clear2 : simulink/Logic and Bit Operations/Bit Clear  iBit=3
  Bit Set : simulink/Logic and Bit Operations/Bit Set  iBit=4
  Bit Set1 : simulink/Logic and Bit Operations/Bit Set  iBit=3
  Bit Set2 : simulink/Logic and Bit Operations/Bit Set  iBit=3
  Bit Set4 : simulink/Logic and Bit Operations/Bit Set  iBit=7
  Constant7 : Constant  Value=0  OutDataTypeStr=boolean
  Delay2 : Delay  DelayLength=1  InitialCondition=1
  Delay3 : Delay  DelayLength=1  InitialCondition=0
  Switch2 : Switch  Criteria=u2 ~= 0
  Switch3 : Switch  Criteria=u2 ~= 0
  Switch4 : Switch  Criteria=u2 ~= 0
  Dfc_id : Outport  OutDataTypeStr=uint8
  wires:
  Dfc_id_nv/1 -> Bit Clear2/1, Bit Set4/1, Bit Clear1/1
  Bit Set4/1 -> Bit Set/1
  Constant7/1 -> Delay2/1
  Delay2/1 -> Switch2/2
  Switch3/1 -> Switch2/3
  Bit Clear2/1 -> Switch2/1
  Switch2/1 -> Delay3/1, Dfc_id/1
  Bit Set1/1 -> Switch3/1
  Bit Set/1 -> Bit Set1/1
  Switch4/1 -> Switch3/3
  Err/1 -> Switch3/2
  Bit Set2/1 -> Switch4/1
  Bit Clear1/1 -> Bit Set2/1
  Delay3/1 -> Switch4/3
  Heal/1 -> Switch4/2

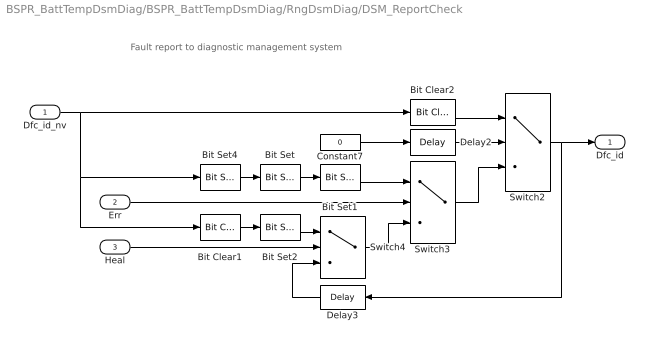
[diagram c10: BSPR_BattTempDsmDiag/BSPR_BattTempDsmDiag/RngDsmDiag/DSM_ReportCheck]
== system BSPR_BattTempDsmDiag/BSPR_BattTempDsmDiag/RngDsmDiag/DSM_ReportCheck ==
  note: Fault report to diagnostic management system
  Dfc_id_nv : Inport  OutDataTypeStr=uint8
  Err : Inport  Port=2
  Heal : Inport  Port=3
  Bit Clear1 : simulink/Logic and Bit Operations/Bit Clear  iBit=4
  Bit Clear2 : simulink/Logic and Bit Operations/Bit Clear  iBit=3
  Bit Set : simulink/Logic and Bit Operations/Bit Set  iBit=4
  Bit Set1 : simulink/Logic and Bit Operations/Bit Set  iBit=3
  Bit Set2 : simulink/Logic and Bit Operations/Bit Set  iBit=3
  Bit Set4 : simulink/Logic and Bit Operations/Bit Set  iBit=7
  Constant7 : Constant  Value=0  OutDataTypeStr=boolean
  Delay2 : Delay  DelayLength=1  InitialCondition=1
  Delay3 : Delay  DelayLength=1  InitialCondition=0
  Switch2 : Switch  Criteria=u2 ~= 0
  Switch3 : Switch  Criteria=u2 ~= 0
  Switch4 : Switch  Criteria=u2 ~= 0
  Dfc_id : Outport  OutDataTypeStr=uint8
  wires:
  Dfc_id_nv/1 -> Bit Clear2/1, Bit Set4/1, Bit Clear1/1
  Bit Set4/1 -> Bit Set/1
  Constant7/1 -> Delay2/1
  Delay2/1 -> Switch2/2
  Switch3/1 -> Switch2/3
  Bit Clear2/1 -> Switch2/1
  Switch2/1 -> Delay3/1, Dfc_id/1
  Bit Set1/1 -> Switch3/1
  Bit Set/1 -> Bit Set1/1
  Switch4/1 -> Switch3/3
  Err/1 -> Switch3/2
  Bit Set2/1 -> Switch4/1
  Bit Clear1/1 -> Bit Set2/1
  Delay3/1 -> Switch4/3
  Heal/1 -> Switch4/2

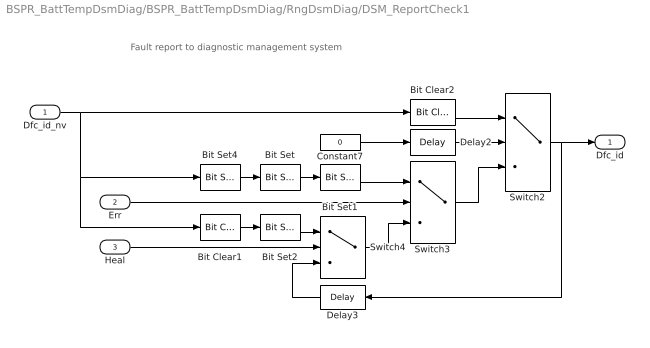
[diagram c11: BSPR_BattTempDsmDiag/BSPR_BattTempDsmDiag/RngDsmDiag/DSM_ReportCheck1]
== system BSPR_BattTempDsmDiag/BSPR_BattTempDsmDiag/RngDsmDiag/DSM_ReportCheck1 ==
  note: Fault report to diagnostic management system
  Dfc_id_nv : Inport  OutDataTypeStr=uint8
  Err : Inport  Port=2
  Heal : Inport  Port=3
  Bit Clear1 : simulink/Logic and Bit Operations/Bit Clear  iBit=4
  Bit Clear2 : simulink/Logic and Bit Operations/Bit Clear  iBit=3
  Bit Set : simulink/Logic and Bit Operations/Bit Set  iBit=4
  Bit Set1 : simulink/Logic and Bit Operations/Bit Set  iBit=3
  Bit Set2 : simulink/Logic and Bit Operations/Bit Set  iBit=3
  Bit Set4 : simulink/Logic and Bit Operations/Bit Set  iBit=7
  Constant7 : Constant  Value=0  OutDataTypeStr=boolean
  Delay2 : Delay  DelayLength=1  InitialCondition=1
  Delay3 : Delay  DelayLength=1  InitialCondition=0
  Switch2 : Switch  Criteria=u2 ~= 0
  Switch3 : Switch  Criteria=u2 ~= 0
  Switch4 : Switch  Criteria=u2 ~= 0
  Dfc_id : Outport  OutDataTypeStr=uint8
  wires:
  Heal/1 -> Switch4/2
  Delay3/1 -> Switch4/3
  Bit Clear1/1 -> Bit Set2/1
  Bit Set2/1 -> Switch4/1
  Err/1 -> Switch3/2
  Switch4/1 -> Switch3/3
  Bit Set/1 -> Bit Set1/1
  Bit Set1/1 -> Switch3/1
  Switch2/1 -> Dfc_id/1, Delay3/1
  Bit Clear2/1 -> Switch2/1
  Switch3/1 -> Switch2/3
  Delay2/1 -> Switch2/2
  Constant7/1 -> Delay2/1
  Bit Set4/1 -> Bit Set/1
  Dfc_id_nv/1 -> Bit Clear1/1, Bit Set4/1, Bit Clear2/1

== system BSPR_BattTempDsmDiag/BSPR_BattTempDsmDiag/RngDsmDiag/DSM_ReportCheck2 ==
  note: Fault report to diagnostic management system
  Dfc_id_nv : Inport  OutDataTypeStr=uint8
  Err : Inport  Port=2
  Heal : Inport  Port=3
  Bit Clear1 : simulink/Logic and Bit Operations/Bit Clear  iBit=4
  Bit Clear2 : simulink/Logic and Bit Operations/Bit Clear  iBit=3
  Bit Set : simulink/Logic and Bit Operations/Bit Set  iBit=4
  Bit Set1 : simulink/Logic and Bit Operations/Bit Set  iBit=3
  Bit Set2 : simulink/Logic and Bit Operations/Bit Set  iBit=3
  Bit Set4 : simulink/Logic and Bit Operations/Bit Set  iBit=7
  Constant7 : Constant  Value=0  OutDataTypeStr=boolean
  Delay2 : Delay  DelayLength=1  InitialCondition=1
  Delay3 : Delay  DelayLength=1  InitialCondition=0
  Switch2 : Switch  Criteria=u2 ~= 0
  Switch3 : Switch  Criteria=u2 ~= 0
  Switch4 : Switch  Criteria=u2 ~= 0
  Dfc_id : Outport  OutDataTypeStr=uint8
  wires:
  Dfc_id_nv/1 -> Bit Clear2/1, Bit Set4/1, Bit Clear1/1
  Bit Set4/1 -> Bit Set/1
  Constant7/1 -> Delay2/1
  Delay2/1 -> Switch2/2
  Switch3/1 -> Switch2/3
  Bit Clear2/1 -> Switch2/1
  Switch2/1 -> Delay3/1, Dfc_id/1
  Bit Set1/1 -> Switch3/1
  Bit Set/1 -> Bit Set1/1
  Switch4/1 -> Switch3/3
  Err/1 -> Switch3/2
  Bit Set2/1 -> Switch4/1
  Bit Clear1/1 -> Bit Set2/1
  Delay3/1 -> Switch4/3
  Heal/1 -> Switch4/2

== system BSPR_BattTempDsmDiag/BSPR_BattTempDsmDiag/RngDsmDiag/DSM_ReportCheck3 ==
  note: Fault report to diagnostic management system
  Dfc_id_nv : Inport  OutDataTypeStr=uint8
  Err : Inport  Port=2
  Heal : Inport  Port=3
  Bit Clear1 : simulink/Logic and Bit Operations/Bit Clear  iBit=4
  Bit Clear2 : simulink/Logic and Bit Operations/Bit Clear  iBit=3
  Bit Set : simulink/Logic and Bit Operations/Bit Set  iBit=4
  Bit Set1 : simulink/Logic and Bit Operations/Bit Set  iBit=3
  Bit Set2 : simulink/Logic and Bit Operations/Bit Set  iBit=3
  Bit Set4 : simulink/Logic and Bit Operations/Bit Set  iBit=7
  Constant7 : Constant  Value=0  OutDataTypeStr=boolean
  Delay2 : Delay  DelayLength=1  InitialCondition=1
  Delay3 : Delay  DelayLength=1  InitialCondition=0
  Switch2 : Switch  Criteria=u2 ~= 0
  Switch3 : Switch  Criteria=u2 ~= 0
  Switch4 : Switch  Criteria=u2 ~= 0
  Dfc_id : Outport  OutDataTypeStr=uint8
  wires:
  Heal/1 -> Switch4/2
  Delay3/1 -> Switch4/3
  Bit Clear1/1 -> Bit Set2/1
  Bit Set2/1 -> Switch4/1
  Err/1 -> Switch3/2
  Switch4/1 -> Switch3/3
  Bit Set/1 -> Bit Set1/1
  Bit Set1/1 -> Switch3/1
  Switch2/1 -> Dfc_id/1, Delay3/1
  Bit Clear2/1 -> Switch2/1
  Switch3/1 -> Switch2/3
  Delay2/1 -> Switch2/2
  Constant7/1 -> Delay2/1
  Bit Set4/1 -> Bit Set/1
  Dfc_id_nv/1 -> Bit Clear1/1, Bit Set4/1, Bit Clear2/1

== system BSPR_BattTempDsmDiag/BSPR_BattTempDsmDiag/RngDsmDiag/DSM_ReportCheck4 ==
  note: Fault report to diagnostic management system
  Dfc_id_nv : Inport  OutDataTypeStr=uint8
  Err : Inport  Port=2
  Heal : Inport  Port=3
  Bit Clear1 : simulink/Logic and Bit Operations/Bit Clear  iBit=4
  Bit Clear2 : simulink/Logic and Bit Operations/Bit Clear  iBit=3
  Bit Set : simulink/Logic and Bit Operations/Bit Set  iBit=4
  Bit Set1 : simulink/Logic and Bit Operations/Bit Set  iBit=3
  Bit Set2 : simulink/Logic and Bit Operations/Bit Set  iBit=3
  Bit Set4 : simulink/Logic and Bit Operations/Bit Set  iBit=7
  Constant7 : Constant  Value=0  OutDataTypeStr=boolean
  Delay2 : Delay  DelayLength=1  InitialCondition=1
  Delay3 : Delay  DelayLength=1  InitialCondition=0
  Switch2 : Switch  Criteria=u2 ~= 0
  Switch3 : Switch  Criteria=u2 ~= 0
  Switch4 : Switch  Criteria=u2 ~= 0
  Dfc_id : Outport  OutDataTypeStr=uint8
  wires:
  Dfc_id_nv/1 -> Bit Clear2/1, Bit Set4/1, Bit Clear1/1
  Bit Set4/1 -> Bit Set/1
  Constant7/1 -> Delay2/1
  Delay2/1 -> Switch2/2
  Switch3/1 -> Switch2/3
  Bit Clear2/1 -> Switch2/1
  Switch2/1 -> Delay3/1, Dfc_id/1
  Bit Set1/1 -> Switch3/1
  Bit Set/1 -> Bit Set1/1
  Switch4/1 -> Switch3/3
  Err/1 -> Switch3/2
  Bit Set2/1 -> Switch4/1
  Bit Clear1/1 -> Bit Set2/1
  Delay3/1 -> Switch4/3
  Heal/1 -> Switch4/2

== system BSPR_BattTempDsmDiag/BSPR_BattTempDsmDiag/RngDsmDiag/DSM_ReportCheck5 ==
  note: Fault report to diagnostic management system
  Dfc_id_nv : Inport  OutDataTypeStr=uint8
  Err : Inport  Port=2
  Heal : Inport  Port=3
  Bit Clear1 : simulink/Logic and Bit Operations/Bit Clear  iBit=4
  Bit Clear2 : simulink/Logic and Bit Operations/Bit Clear  iBit=3
  Bit Set : simulink/Logic and Bit Operations/Bit Set  iBit=4
  Bit Set1 : simulink/Logic and Bit Operations/Bit Set  iBit=3
  Bit Set2 : simulink/Logic and Bit Operations/Bit Set  iBit=3
  Bit Set4 : simulink/Logic and Bit Operations/Bit Set  iBit=7
  Constant7 : Constant  Value=0  OutDataTypeStr=boolean
  Delay2 : Delay  DelayLength=1  InitialCondition=1
  Delay3 : Delay  DelayLength=1  InitialCondition=0
  Switch2 : Switch  Criteria=u2 ~= 0
  Switch3 : Switch  Criteria=u2 ~= 0
  Switch4 : Switch  Criteria=u2 ~= 0
  Dfc_id : Outport  OutDataTypeStr=uint8
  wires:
  Heal/1 -> Switch4/2
  Delay3/1 -> Switch4/3
  Bit Clear1/1 -> Bit Set2/1
  Bit Set2/1 -> Switch4/1
  Err/1 -> Switch3/2
  Switch4/1 -> Switch3/3
  Bit Set/1 -> Bit Set1/1
  Bit Set1/1 -> Switch3/1
  Switch2/1 -> Dfc_id/1, Delay3/1
  Bit Clear2/1 -> Switch2/1
  Switch3/1 -> Switch2/3
  Delay2/1 -> Switch2/2
  Constant7/1 -> Delay2/1
  Bit Set4/1 -> Bit Set/1
  Dfc_id_nv/1 -> Bit Clear1/1, Bit Set4/1, Bit Clear2/1

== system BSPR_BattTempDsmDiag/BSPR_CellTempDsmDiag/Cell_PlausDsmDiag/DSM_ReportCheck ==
  note: Fault report to diagnostic management system
  Dfc_id_nv : Inport  OutDataTypeStr=uint8
  Err : Inport  Port=2
  Heal : Inport  Port=3
  Bit Clear1 : simulink/Logic and Bit Operations/Bit Clear  iBit=4
  Bit Clear2 : simulink/Logic and Bit Operations/Bit Clear  iBit=3
  Bit Set : simulink/Logic and Bit Operations/Bit Set  iBit=4
  Bit Set1 : simulink/Logic and Bit Operations/Bit Set  iBit=3
  Bit Set2 : simulink/Logic and Bit Operations/Bit Set  iBit=3
  Bit Set4 : simulink/Logic and Bit Operations/Bit Set  iBit=7
  Constant7 : Constant  Value=0  OutDataTypeStr=boolean
  Delay2 : Delay  DelayLength=1  InitialCondition=1
  Delay3 : Delay  DelayLength=1  InitialCondition=0
  Switch2 : Switch  Criteria=u2 ~= 0
  Switch3 : Switch  Criteria=u2 ~= 0
  Switch4 : Switch  Criteria=u2 ~= 0
  Dfc_id : Outport  OutDataTypeStr=uint8
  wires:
  Heal/1 -> Switch4/2
  Delay3/1 -> Switch4/3
  Bit Clear1/1 -> Bit Set2/1
  Bit Set2/1 -> Switch4/1
  Err/1 -> Switch3/2
  Switch4/1 -> Switch3/3
  Bit Set/1 -> Bit Set1/1
  Bit Set1/1 -> Switch3/1
  Switch2/1 -> Dfc_id/1, Delay3/1
  Bit Clear2/1 -> Switch2/1
  Switch3/1 -> Switch2/3
  Delay2/1 -> Switch2/2
  Constant7/1 -> Delay2/1
  Bit Set4/1 -> Bit Set/1
  Dfc_id_nv/1 -> Bit Clear1/1, Bit Set4/1, Bit Clear2/1

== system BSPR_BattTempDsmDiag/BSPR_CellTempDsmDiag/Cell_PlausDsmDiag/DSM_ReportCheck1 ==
  note: Fault report to diagnostic management system
  Dfc_id_nv : Inport  OutDataTypeStr=uint8
  Err : Inport  Port=2
  Heal : Inport  Port=3
  Bit Clear1 : simulink/Logic and Bit Operations/Bit Clear  iBit=4
  Bit Clear2 : simulink/Logic and Bit Operations/Bit Clear  iBit=3
  Bit Set : simulink/Logic and Bit Operations/Bit Set  iBit=4
  Bit Set1 : simulink/Logic and Bit Operations/Bit Set  iBit=3
  Bit Set2 : simulink/Logic and Bit Operations/Bit Set  iBit=3
  Bit Set4 : simulink/Logic and Bit Operations/Bit Set  iBit=7
  Constant7 : Constant  Value=0  OutDataTypeStr=boolean
  Delay2 : Delay  DelayLength=1  InitialCondition=1
  Delay3 : Delay  DelayLength=1  InitialCondition=0
  Switch2 : Switch  Criteria=u2 ~= 0
  Switch3 : Switch  Criteria=u2 ~= 0
  Switch4 : Switch  Criteria=u2 ~= 0
  Dfc_id : Outport  OutDataTypeStr=uint8
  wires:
  Dfc_id_nv/1 -> Bit Clear2/1, Bit Set4/1, Bit Clear1/1
  Bit Set4/1 -> Bit Set/1
  Constant7/1 -> Delay2/1
  Delay2/1 -> Switch2/2
  Switch3/1 -> Switch2/3
  Bit Clear2/1 -> Switch2/1
  Switch2/1 -> Delay3/1, Dfc_id/1
  Bit Set1/1 -> Switch3/1
  Bit Set/1 -> Bit Set1/1
  Switch4/1 -> Switch3/3
  Err/1 -> Switch3/2
  Bit Set2/1 -> Switch4/1
  Bit Clear1/1 -> Bit Set2/1
  Delay3/1 -> Switch4/3
  Heal/1 -> Switch4/2

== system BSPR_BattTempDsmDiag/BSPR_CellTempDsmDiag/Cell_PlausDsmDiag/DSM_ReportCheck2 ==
  note: Fault report to diagnostic management system
  Dfc_id_nv : Inport  OutDataTypeStr=uint8
  Err : Inport  Port=2
  Heal : Inport  Port=3
  Bit Clear1 : simulink/Logic and Bit Operations/Bit Clear  iBit=4
  Bit Clear2 : simulink/Logic and Bit Operations/Bit Clear  iBit=3
  Bit Set : simulink/Logic and Bit Operations/Bit Set  iBit=4
  Bit Set1 : simulink/Logic and Bit Operations/Bit Set  iBit=3
  Bit Set2 : simulink/Logic and Bit Operations/Bit Set  iBit=3
  Bit Set4 : simulink/Logic and Bit Operations/Bit Set  iBit=7
  Constant7 : Constant  Value=0  OutDataTypeStr=boolean
  Delay2 : Delay  DelayLength=1  InitialCondition=1
  Delay3 : Delay  DelayLength=1  InitialCondition=0
  Switch2 : Switch  Criteria=u2 ~= 0
  Switch3 : Switch  Criteria=u2 ~= 0
  Switch4 : Switch  Criteria=u2 ~= 0
  Dfc_id : Outport  OutDataTypeStr=uint8
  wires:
  Heal/1 -> Switch4/2
  Delay3/1 -> Switch4/3
  Bit Clear1/1 -> Bit Set2/1
  Bit Set2/1 -> Switch4/1
  Err/1 -> Switch3/2
  Switch4/1 -> Switch3/3
  Bit Set/1 -> Bit Set1/1
  Bit Set1/1 -> Switch3/1
  Switch2/1 -> Dfc_id/1, Delay3/1
  Bit Clear2/1 -> Switch2/1
  Switch3/1 -> Switch2/3
  Delay2/1 -> Switch2/2
  Constant7/1 -> Delay2/1
  Bit Set4/1 -> Bit Set/1
  Dfc_id_nv/1 -> Bit Clear1/1, Bit Set4/1, Bit Clear2/1

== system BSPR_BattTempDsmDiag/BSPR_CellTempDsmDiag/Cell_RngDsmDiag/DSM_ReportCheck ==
  note: Fault report to diagnostic management system
  Dfc_id_nv : Inport  OutDataTypeStr=uint8
  Err : Inport  Port=2
  Heal : Inport  Port=3
  Bit Clear1 : simulink/Logic and Bit Operations/Bit Clear  iBit=4
  Bit Clear2 : simulink/Logic and Bit Operations/Bit Clear  iBit=3
  Bit Set : simulink/Logic and Bit Operations/Bit Set  iBit=4
  Bit Set1 : simulink/Logic and Bit Operations/Bit Set  iBit=3
  Bit Set2 : simulink/Logic and Bit Operations/Bit Set  iBit=3
  Bit Set4 : simulink/Logic and Bit Operations/Bit Set  iBit=7
  Constant7 : Constant  Value=0  OutDataTypeStr=boolean
  Delay2 : Delay  DelayLength=1  InitialCondition=1
  Delay3 : Delay  DelayLength=1  InitialCondition=0
  Switch2 : Switch  Criteria=u2 ~= 0
  Switch3 : Switch  Criteria=u2 ~= 0
  Switch4 : Switch  Criteria=u2 ~= 0
  Dfc_id : Outport  OutDataTypeStr=uint8
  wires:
  Heal/1 -> Switch4/2
  Delay3/1 -> Switch4/3
  Bit Clear1/1 -> Bit Set2/1
  Bit Set2/1 -> Switch4/1
  Err/1 -> Switch3/2
  Switch4/1 -> Switch3/3
  Bit Set/1 -> Bit Set1/1
  Bit Set1/1 -> Switch3/1
  Switch2/1 -> Dfc_id/1, Delay3/1
  Bit Clear2/1 -> Switch2/1
  Switch3/1 -> Switch2/3
  Delay2/1 -> Switch2/2
  Constant7/1 -> Delay2/1
  Bit Set4/1 -> Bit Set/1
  Dfc_id_nv/1 -> Bit Clear1/1, Bit Set4/1, Bit Clear2/1

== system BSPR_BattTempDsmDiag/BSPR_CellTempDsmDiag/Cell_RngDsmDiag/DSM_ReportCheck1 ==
  note: Fault report to diagnostic management system
  Dfc_id_nv : Inport  OutDataTypeStr=uint8
  Err : Inport  Port=2
  Heal : Inport  Port=3
  Bit Clear1 : simulink/Logic and Bit Operations/Bit Clear  iBit=4
  Bit Clear2 : simulink/Logic and Bit Operations/Bit Clear  iBit=3
  Bit Set : simulink/Logic and Bit Operations/Bit Set  iBit=4
  Bit Set1 : simulink/Logic and Bit Operations/Bit Set  iBit=3
  Bit Set2 : simulink/Logic and Bit Operations/Bit Set  iBit=3
  Bit Set4 : simulink/Logic and Bit Operations/Bit Set  iBit=7
  Constant7 : Constant  Value=0  OutDataTypeStr=boolean
  Delay2 : Delay  DelayLength=1  InitialCondition=1
  Delay3 : Delay  DelayLength=1  InitialCondition=0
  Switch2 : Switch  Criteria=u2 ~= 0
  Switch3 : Switch  Criteria=u2 ~= 0
  Switch4 : Switch  Criteria=u2 ~= 0
  Dfc_id : Outport  OutDataTypeStr=uint8
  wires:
  Dfc_id_nv/1 -> Bit Clear2/1, Bit Set4/1, Bit Clear1/1
  Bit Set4/1 -> Bit Set/1
  Constant7/1 -> Delay2/1
  Delay2/1 -> Switch2/2
  Switch3/1 -> Switch2/3
  Bit Clear2/1 -> Switch2/1
  Switch2/1 -> Delay3/1, Dfc_id/1
  Bit Set1/1 -> Switch3/1
  Bit Set/1 -> Bit Set1/1
  Switch4/1 -> Switch3/3
  Err/1 -> Switch3/2
  Bit Set2/1 -> Switch4/1
  Bit Clear1/1 -> Bit Set2/1
  Delay3/1 -> Switch4/3
  Heal/1 -> Switch4/2

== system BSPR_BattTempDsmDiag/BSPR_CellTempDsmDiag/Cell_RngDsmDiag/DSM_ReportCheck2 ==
  note: Fault report to diagnostic management system
  Dfc_id_nv : Inport  OutDataTypeStr=uint8
  Err : Inport  Port=2
  Heal : Inport  Port=3
  Bit Clear1 : simulink/Logic and Bit Operations/Bit Clear  iBit=4
  Bit Clear2 : simulink/Logic and Bit Operations/Bit Clear  iBit=3
  Bit Set : simulink/Logic and Bit Operations/Bit Set  iBit=4
  Bit Set1 : simulink/Logic and Bit Operations/Bit Set  iBit=3
  Bit Set2 : simulink/Logic and Bit Operations/Bit Set  iBit=3
  Bit Set4 : simulink/Logic and Bit Operations/Bit Set  iBit=7
  Constant7 : Constant  Value=0  OutDataTypeStr=boolean
  Delay2 : Delay  DelayLength=1  InitialCondition=1
  Delay3 : Delay  DelayLength=1  InitialCondition=0
  Switch2 : Switch  Criteria=u2 ~= 0
  Switch3 : Switch  Criteria=u2 ~= 0
  Switch4 : Switch  Criteria=u2 ~= 0
  Dfc_id : Outport  OutDataTypeStr=uint8
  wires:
  Heal/1 -> Switch4/2
  Delay3/1 -> Switch4/3
  Bit Clear1/1 -> Bit Set2/1
  Bit Set2/1 -> Switch4/1
  Err/1 -> Switch3/2
  Switch4/1 -> Switch3/3
  Bit Set/1 -> Bit Set1/1
  Bit Set1/1 -> Switch3/1
  Switch2/1 -> Dfc_id/1, Delay3/1
  Bit Clear2/1 -> Switch2/1
  Switch3/1 -> Switch2/3
  Delay2/1 -> Switch2/2
  Constant7/1 -> Delay2/1
  Bit Set4/1 -> Bit Set/1
  Dfc_id_nv/1 -> Bit Clear1/1, Bit Set4/1, Bit Clear2/1

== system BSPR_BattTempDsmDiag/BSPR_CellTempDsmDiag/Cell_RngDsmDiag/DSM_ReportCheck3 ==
  note: Fault report to diagnostic management system
  Dfc_id_nv : Inport  OutDataTypeStr=uint8
  Err : Inport  Port=2
  Heal : Inport  Port=3
  Bit Clear1 : simulink/Logic and Bit Operations/Bit Clear  iBit=4
  Bit Clear2 : simulink/Logic and Bit Operations/Bit Clear  iBit=3
  Bit Set : simulink/Logic and Bit Operations/Bit Set  iBit=4
  Bit Set1 : simulink/Logic and Bit Operations/Bit Set  iBit=3
  Bit Set2 : simulink/Logic and Bit Operations/Bit Set  iBit=3
  Bit Set4 : simulink/Logic and Bit Operations/Bit Set  iBit=7
  Constant7 : Constant  Value=0  OutDataTypeStr=boolean
  Delay2 : Delay  DelayLength=1  InitialCondition=1
  Delay3 : Delay  DelayLength=1  InitialCondition=0
  Switch2 : Switch  Criteria=u2 ~= 0
  Switch3 : Switch  Criteria=u2 ~= 0
  Switch4 : Switch  Criteria=u2 ~= 0
  Dfc_id : Outport  OutDataTypeStr=uint8
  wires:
  Dfc_id_nv/1 -> Bit Clear2/1, Bit Set4/1, Bit Clear1/1
  Bit Set4/1 -> Bit Set/1
  Constant7/1 -> Delay2/1
  Delay2/1 -> Switch2/2
  Switch3/1 -> Switch2/3
  Bit Clear2/1 -> Switch2/1
  Switch2/1 -> Delay3/1, Dfc_id/1
  Bit Set1/1 -> Switch3/1
  Bit Set/1 -> Bit Set1/1
  Switch4/1 -> Switch3/3
  Err/1 -> Switch3/2
  Bit Set2/1 -> Switch4/1
  Bit Clear1/1 -> Bit Set2/1
  Delay3/1 -> Switch4/3
  Heal/1 -> Switch4/2

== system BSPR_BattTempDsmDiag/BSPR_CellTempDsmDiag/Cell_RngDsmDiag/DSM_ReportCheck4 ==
  note: Fault report to diagnostic management system
  Dfc_id_nv : Inport  OutDataTypeStr=uint8
  Err : Inport  Port=2
  Heal : Inport  Port=3
  Bit Clear1 : simulink/Logic and Bit Operations/Bit Clear  iBit=4
  Bit Clear2 : simulink/Logic and Bit Operations/Bit Clear  iBit=3
  Bit Set : simulink/Logic and Bit Operations/Bit Set  iBit=4
  Bit Set1 : simulink/Logic and Bit Operations/Bit Set  iBit=3
  Bit Set2 : simulink/Logic and Bit Operations/Bit Set  iBit=3
  Bit Set4 : simulink/Logic and Bit Operations/Bit Set  iBit=7
  Constant7 : Constant  Value=0  OutDataTypeStr=boolean
  Delay2 : Delay  DelayLength=1  InitialCondition=1
  Delay3 : Delay  DelayLength=1  InitialCondition=0
  Switch2 : Switch  Criteria=u2 ~= 0
  Switch3 : Switch  Criteria=u2 ~= 0
  Switch4 : Switch  Criteria=u2 ~= 0
  Dfc_id : Outport  OutDataTypeStr=uint8
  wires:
  Heal/1 -> Switch4/2
  Delay3/1 -> Switch4/3
  Bit Clear1/1 -> Bit Set2/1
  Bit Set2/1 -> Switch4/1
  Err/1 -> Switch3/2
  Switch4/1 -> Switch3/3
  Bit Set/1 -> Bit Set1/1
  Bit Set1/1 -> Switch3/1
  Switch2/1 -> Dfc_id/1, Delay3/1
  Bit Clear2/1 -> Switch2/1
  Switch3/1 -> Switch2/3
  Delay2/1 -> Switch2/2
  Constant7/1 -> Delay2/1
  Bit Set4/1 -> Bit Set/1
  Dfc_id_nv/1 -> Bit Clear1/1, Bit Set4/1, Bit Clear2/1

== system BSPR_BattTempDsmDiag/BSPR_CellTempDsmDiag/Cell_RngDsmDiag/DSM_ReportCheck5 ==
  note: Fault report to diagnostic management system
  Dfc_id_nv : Inport  OutDataTypeStr=uint8
  Err : Inport  Port=2
  Heal : Inport  Port=3
  Bit Clear1 : simulink/Logic and Bit Operations/Bit Clear  iBit=4
  Bit Clear2 : simulink/Logic and Bit Operations/Bit Clear  iBit=3
  Bit Set : simulink/Logic and Bit Operations/Bit Set  iBit=4
  Bit Set1 : simulink/Logic and Bit Operations/Bit Set  iBit=3
  Bit Set2 : simulink/Logic and Bit Operations/Bit Set  iBit=3
  Bit Set4 : simulink/Logic and Bit Operations/Bit Set  iBit=7
  Constant7 : Constant  Value=0  OutDataTypeStr=boolean
  Delay2 : Delay  DelayLength=1  InitialCondition=1
  Delay3 : Delay  DelayLength=1  InitialCondition=0
  Switch2 : Switch  Criteria=u2 ~= 0
  Switch3 : Switch  Criteria=u2 ~= 0
  Switch4 : Switch  Criteria=u2 ~= 0
  Dfc_id : Outport  OutDataTypeStr=uint8
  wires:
  Dfc_id_nv/1 -> Bit Clear2/1, Bit Set4/1, Bit Clear1/1
  Bit Set4/1 -> Bit Set/1
  Constant7/1 -> Delay2/1
  Delay2/1 -> Switch2/2
  Switch3/1 -> Switch2/3
  Bit Clear2/1 -> Switch2/1
  Switch2/1 -> Delay3/1, Dfc_id/1
  Bit Set1/1 -> Switch3/1
  Bit Set/1 -> Bit Set1/1
  Switch4/1 -> Switch3/3
  Err/1 -> Switch3/2
  Bit Set2/1 -> Switch4/1
  Bit Clear1/1 -> Bit Set2/1
  Delay3/1 -> Switch4/3
  Heal/1 -> Switch4/2
